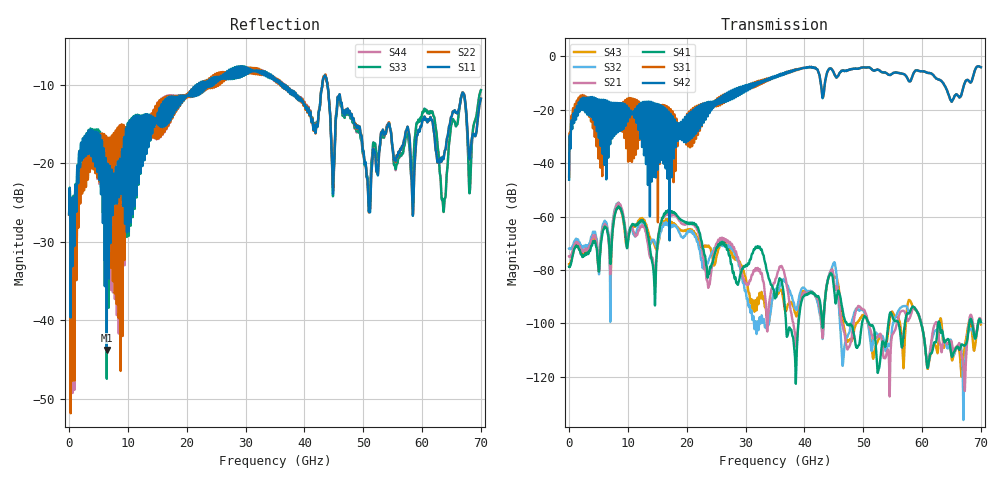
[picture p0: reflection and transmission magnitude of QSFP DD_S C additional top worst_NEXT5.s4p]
! AWR Design Environment (8415) Fri Dec 21 09:08:24 2018
! Document = 'CHANNEL TEST'
! nPorts: 4, nXvals: 7001
# HZ S DB R 50
!Freq DBS11 AngS11 DBS12 AngS12 DBS13 AngS13 DBS14 AngS14
!	DBS21 AngS21 DBS22 AngS22 DBS23 AngS23 DBS24 AngS24
!	DBS31 AngS31 DBS32 AngS32 DBS33 AngS33 DBS34 AngS34
!	DBS41 AngS41 DBS42 AngS42 DBS43 AngS43 DBS44 AngS44
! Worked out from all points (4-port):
!   7000 points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, 10 MHz to 70 GHz, reference 50 ohm
!   strongest paths, dB at 10 MHz, 17.51 GHz, 35.01 GHz, 52.51 GHz, 70 GHz:
!     S42: -46.2, -25.1, -7.4, -5.0, -4.0
!     S31: -45.1, -23.1, -7.6, -5.0, -4.0
!     S41: -78.8, -58.0, -90.6, -118.2, -99.4
!     S21: -74.9, -59.1, -84.3, -104.8, -98.6
!     S32: -71.9, -63.3, -87.8, -104.1, -99.6
!     S43: -77.8, -62.2, -88.8, -106.3, -100.4
!   lowest |S11| = -43.8 dB at 6.41 GHz (marker M1), VSWR 1.01, Z = 50.5 - j0.428 ohm
!   |S11| at or under -10 dB: start of sweep to 21.78 GHz; 36.52 GHz to 43.04 GHz (6.515 GHz wide, 16.4 % of centre); 43.91 GHz to end of sweep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
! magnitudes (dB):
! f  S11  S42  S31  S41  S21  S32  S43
! 10 MHz  -26.5  -46.2  -45.1  -78.8  -74.9  -71.9  -77.8
! 1.65 GHz  -19.9  -17.2  -15.4  -72.1  -70.7  -69.4  -71.9
! 6.41 GHz  -43.8  -20.6  -18.7  -64.5  -63.9  -62.8  -63.5
! 17.8 GHz  -13.0  -32.4  -29.5  -58.3  -59.1  -63.0  -62.4
! 30.78 GHz  -8.1  -11.1  -11.9  -76.1  -84.0  -95.3  -91.8
! 63.65 GHz  -19.4  -10.2  -10.2  -105.6  -106.0  -105.6  -109.0
! 70 GHz  -11.8  -4.0  -4.0  -99.4  -98.6  -99.6  -100.4
